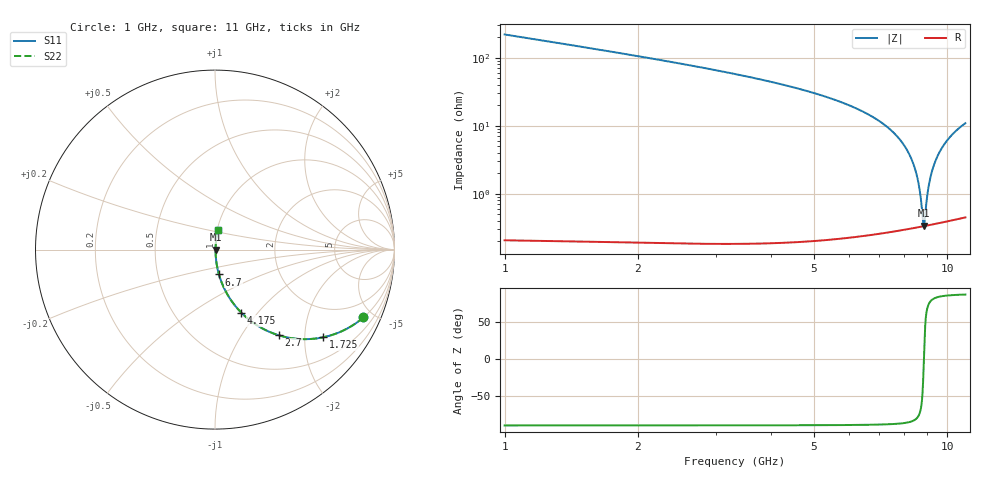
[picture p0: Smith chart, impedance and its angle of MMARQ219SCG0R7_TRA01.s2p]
! MMARQ219SCG0R7_TRA01  S-PARAMETER MODEL  ( General Type )
! Model Generated by TAIYO YUDEN Corporation (http://www.ty-top.com)
! Version 1.0
! TAIYO YUDEN Control No. 160201
! Copyright(c) 2016 TAIYO YUDEN CO.,LTD. All Rights Reserved.
! Product Description (link to TY-COMPAS)
! https://ds.yuden.co.jp/TYCOMPAS/or/detail?pn=MMARQ219SCG0R7BTRA01&u=M
! Products Name : Multilayer Ceramic Capacitors
! Characteristics :
!  Capacitance : 0.7 pF , Rated Voltage : 250V , TCC : CG / C0G
!  Case Size : 2.0 x 1.25 / 0.079 x 0.049 [mm/inch] , Thickness : 0.85 / 0.033 [mm/inch]
!  (Conditions: Temperature = 25 degC , DC Bias Current/Voltage = 0A / 0V)
! External Node Assignments :
!  1  o---| |---o  2
! GND o---------o GND
! Frequency Range : 1000MHz  -  11000MHz  [ 401 STEP ]
# MHz S RI R 50
! Freq[MHz].  S11 Real  S11 Imag  S21 Real  S21 Imag  S12 Real  S12 Imag  S22 Real  S22 Imag
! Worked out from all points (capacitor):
!   401 points, 1 GHz to 11 GHz, reference 50 ohm
!   read as one part in series: C = 718 fF near 1.05 GHz
!   lowest |Z| = 341 mohm at 8.85 GHz (marker M1)
!   series resonance near 8.862 GHz, so ESL is about 450 pH
!   S11 on the Smith chart (normalised r, x): 1 GHz: 1.00, -4.37; 1.725 GHz: 1.00, -2.47; 2.7 GHz: 1.00, -1.49; 4.175 GHz: 1.00, -0.83; 6.7 GHz: 1.00, -0.28; 11 GHz: 1.01, +0.22
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1000  0.8269 -0.3779  0.1731 0.3779  0.1731 0.3779  0.8269 -0.3779
1725  0.6041 -0.4882  0.3959 0.4882  0.3959 0.4882  0.6041 -0.4882
2675  0.3622 -0.4794  0.6378 0.4794  0.6378 0.4794  0.3622 -0.4794
2700  0.357 -0.4779  0.643 0.4779  0.643 0.4779  0.357 -0.4779
4175  0.1469 -0.3517  0.8531 0.3517  0.8531 0.3517  0.1469 -0.3517
4350  0.1314 -0.3353  0.8686 0.3353  0.8686 0.3353  0.1314 -0.3353
6000  0.0405 -0.1916  0.9595 0.1916  0.9595 0.1916  0.0405 -0.1916
6700  0.022 -0.1383  0.978 0.1383  0.978 0.1383  0.022 -0.1383
7675  0.00797 -0.0714  0.992 0.0714  0.992 0.0714  0.00797 -0.0714
8125  0.00488 -0.0431  0.9951 0.0431  0.9951 0.0431  0.00488 -0.0431
8450  0.00371 -0.0237  0.9963 0.0237  0.9963 0.0237  0.00371 -0.0237
8650  0.00339 -0.012  0.9966 0.012  0.9966 0.012  0.00339 -0.012
8725  0.00334 -0.00773  0.9967 0.00773  0.9967 0.00773  0.00334 -0.00773
8825  0.00333 -0.00207  0.9967 0.00207  0.9967 0.00207  0.00333 -0.00207
8850  0.00334 -0.000662  0.9967 0.000662  0.9967 0.000662  0.00334 -0.000662
8900  0.00337 0.00214  0.9966 -0.00214  0.9966 -0.00214  0.00337 0.00214
9000  0.00347 0.00769  0.9965 -0.00769  0.9965 -0.00769  0.00347 0.00769
9100  0.00363 0.0132  0.9964 -0.0132  0.9964 -0.0132  0.00363 0.0132
9350  0.00429 0.0266  0.9957 -0.0266  0.9957 -0.0266  0.00429 0.0266
9625  0.00541 0.041  0.9946 -0.041  0.9946 -0.041  0.00541 0.041
9975  0.00737 0.0587  0.9926 -0.0587  0.9926 -0.0587  0.00737 0.0587
11000  0.0161 0.1067  0.9839 -0.1067  0.9839 -0.1067  0.0161 0.1067
